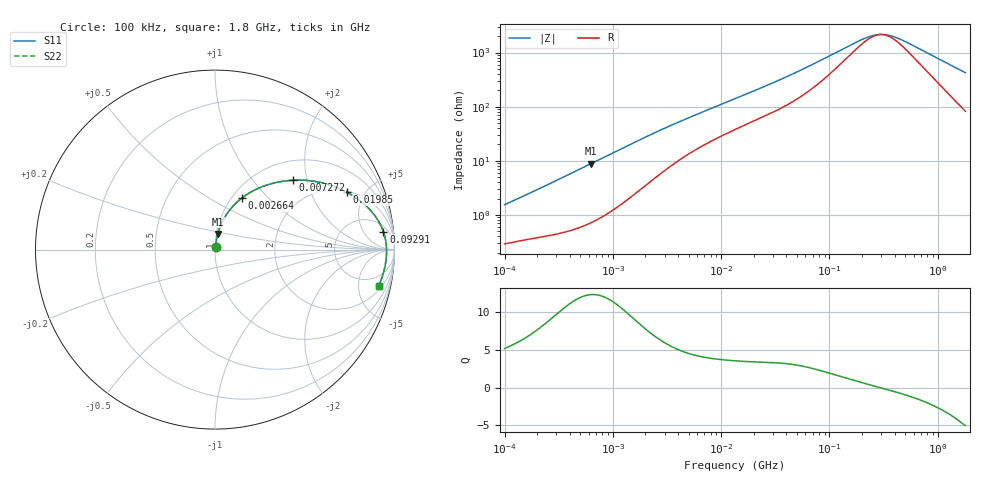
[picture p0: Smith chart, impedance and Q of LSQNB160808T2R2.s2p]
! LSQNB160808T2R2  S-PARAMETER MODEL  ( General Type )
! Model Generated by TAIYO YUDEN Corporation (http://www.ty-top.com)
! Version 3.0
! TAIYO YUDEN Control No. 100810NG19SB-FKC
! Copyright(c) 2007 TAIYO YUDEN CO.,LTD. All Rights Reserved.
! Product Description (link to TY-COMPAS)
! https://ds.yuden.co.jp/TYCOMPAS/or/detail?pn=LSQNB160808T2R2M&u=M
! Products Name : Inductors
! Characteristics :
!  Inductance : 2.2 uH , SRF(min) : 80 MHz , DC Resistance(max) : 0.221 Ohm
!  Rated Current : Saturation :190 mA , Temp Rise : 560 mA (40 degC)
!  Case Size : 1.6 x 0.8 / 0.063 x 0.031 [mm/inch] , Thickness : 0.8 / 0.031 [mm/inch]
!  (Conditions: Temperature = 25 degC , DC Bias Current/Voltage = 0A / 0V)
! External Node Assignments :
!  1  o---GGG---o  2
! GND o---------o GND
! Frequency Range : 0.1MHz  -  1800MHz  [ 402 STEP ]
# MHz S RI R 50
! Freq[MHz].  S11 Real  S11 Imag  S21 Real  S21 Imag  S12 Real  S12 Imag  S22 Real  S22 Imag
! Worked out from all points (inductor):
!   401 points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, 100 kHz to 1.8 GHz, reference 50 ohm
!   read as one part in series: L = 2.36 uH near 105 kHz
!   highest Q = 12.4 at 627.9 kHz (marker M1), where L = 2.24 uH
!   self-resonance near 297.9 MHz
!   S11 on the Smith chart (normalised r, x): 100 kHz: 1.01, +0.03; 2.664 MHz: 1.11, +0.71; 7.272 MHz: 1.41, +1.65; 19.85 MHz: 2.08, +3.72; 92.91 MHz: 8, +14; 1.8 GHz: 2.64, -8.34
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0.1  0.00312 0.0151  0.9969 -0.0151  0.9969 -0.0151  0.00312 0.0151
0.253659  0.00541 0.0361  0.9946 -0.0361  0.9946 -0.0361  0.00541 0.0361
0.516129  0.0112 0.0717  0.9888 -0.0717  0.9888 -0.0717  0.0112 0.0717
0.627861  0.0147 0.0865  0.9853 -0.0865  0.9853 -0.0865  0.0147 0.0865
1.409041  0.0542 0.1808  0.9458 -0.1808  0.9458 -0.1808  0.0542 0.1808
1.937403  0.0914 0.2322  0.9086 -0.2322  0.9086 -0.2322  0.0914 0.2322
2.66389  0.1478 0.2859  0.8522 -0.2859  0.8522 -0.2859  0.1478 0.2859
4.566214  0.2874 0.3593  0.7126 -0.3593  0.7126 -0.3593  0.2874 0.3593
7.272466  0.4349 0.3865  0.5651 -0.3865  0.5651 -0.3865  0.4349 0.3865
13.41641  0.63 0.3629  0.37 -0.3629  0.37 -0.3629  0.63 0.3629
19.85396  0.7359 0.3189  0.2641 -0.3189  0.2641 -0.3189  0.7359 0.3189
36.62703  0.8567 0.229  0.1433 -0.229  0.1433 -0.229  0.8567 0.229
69.24595  0.9231 0.1356  0.0769 -0.1356  0.0769 -0.1356  0.9231 0.1356
92.90788  0.9381 0.0997  0.0619 -0.0997  0.0619 -0.0997  0.9381 0.0997
175.6488  0.9526 0.0394  0.0474 -0.0394  0.0474 -0.0394  0.9526 0.0394
229.9669  0.9548 0.0187  0.0452 -0.0187  0.0452 -0.0187  0.9548 0.0187
286.6876  0.9556 0.00275  0.0444 -0.00275  0.0444 -0.00275  0.9556 0.00275
357.3983  0.9558 -0.0131  0.0442 0.0131  0.0442 0.0131  0.9558 -0.0131
413.9822  0.9555 -0.024  0.0445 0.024  0.0445 0.024  0.9555 -0.024
491.4156  0.9548 -0.0374  0.0452 0.0374  0.0452 0.0374  0.9548 -0.0374
975.7037  0.9447 -0.1054  0.0553 0.1054  0.0553 0.1054  0.9447 -0.1054
1800  0.9119 -0.2014  0.0881 0.2014  0.0881 0.2014  0.9119 -0.2014
